(* Logix 5000 AddOnInstructionDefinition export Banner_IOLM_T_v2_2; software revision 32.00 *)

TYPE Banner_IOL_Port_v2 :   // UDT that has all of the data items necessary to communicate with a specific Port on a IO-Link Master
STRUCT
   Port_Controlled : INT;   // Each bit represents a port on an IO-Link Master. Set to 1 to tell AOI to control that port.
   Port_Activate : INT;   // Each bit represents a port on an IO-Link Master. When ON that port will process any commands in queue.
   Port_Read : INT;   // Each bit represents a port on an IO-Link Master. Used to determine when device AOI has requested a Read command.
   Port_Write : INT;   // Each bit represents a port on an IO-Link Master. Used to determine when device AOI has requested a Write command.
   Port_RW_Complete : INT;   // Each bit represents a port on an IO-Link Master. Tells device AOI that Read or Write request has been completed.
   Port_Device_Read : INT;
   Data_Transfer : SINT[70];   // Array to transfer data from IO-Master to device AOIs.
END_STRUCT
END_TYPE

TYPE Banner_IOLM_EL_v2 :   // Error Log for Messages to IOLM.
STRUCT
   RW : SINT;   // 0 = Read, 1 = Write.
   Port : SINT;   // Port number that generated error.
   Index : SINT;   // IO-Link Index for generated error.
END_STRUCT
END_TYPE

TYPE Banner_IOLM_v2 :   // UDT to control IO-Link Masters.
STRUCT
   Message_Source_Data : SINT[70];   // Array used to generate the source data for an Explicit Message
   Message_Destination_Data : SINT[70];   // Array that stores the data from the IO-Link sensor for an Explicit Message.
   Error_Log : Banner_IOLM_EL_v2[10];
   Error_Write_Retry : BOOL;
   Num_Error_MSGS : DINT;
   IO_Link_Master_Busy : BOOL;   // 0 = While waiting for a command, 1 = Processing command
   AOI_Reset : BOOL;
   Port_Data : Banner_IOL_Port_v2;   // All of the necessary data to work with the various ports of the IO-Link Master.
   Halt_Operation : BOOL;   // When parameter is 1 the AOI is halted as next available time frame.
   AOI_Halted : BOOL;   // AOI is in standby mode until Halt Operation tag is set back to 0.
END_STRUCT
END_TYPE

TYPE IOLRequest :
STRUCT
   Enable_Multiple_Nodes : BOOL; {access None}   // Set to 1 to enable multiple nodes
   ApplicationPath : STRING; {access None}   // Set Path for following IOL Instructions
   Read : BOOL; {access None}   // For internal use to integrate IOLRead and IOWrite with IOLService
   Write : BOOL; {access None}   // For internal use to integrate IOLRead and IOWrite with IOLService
   Reset : BOOL; {access None}   // For internal use to integrate IOLRead and IOWrite with IOLService
   Done : BOOL; {access None}   // For internal use to integrate IOLRead and IOWrite with IOLService
   Error : BOOL; {access None}   // For internal use to integrate IOLRead and IOWrite with IOLService
   Slot : INT; {access None}   // For internal use to integrate IOLRead and IOWrite with IOLService
   Port : INT; {access None}   // For internal use to integrate IOLRead and IOWrite with IOLService
   Index : INT; {access None}   // For internal use to integrate IOLRead and IOWrite with IOLService
   SubIndex : INT; {access None}   // For internal use to integrate IOLRead and IOWrite with IOLService
   Length : INT; {access None}   // For internal use to integrate IOLRead and IOWrite with IOLService
   Handle : INT; {access None}   // For internal use to integrate IOLRead and IOWrite with IOLService
   Status : INT; {access None}   // For internal use to integrate IOLRead and IOWrite with IOLService
   NextHandle : INT; {access None}   // For internal use to integrate IOLRead and IOWrite with IOLService
   ReceiveData : SINT[145]; {access None}   // For internal use to integrate IOLRead and IOWrite with IOLService
   SendData : SINT[145]; {access None}   // For internal use to integrate IOLRead and IOWrite with IOLService
   WriteData : DINT; {access None}   // For internal use to integrate IOLRead and IOWrite with IOLService
   ActivePath : STRING; {access None}   // For internal use to integrate IOLRead and IOWrite with IOLService
END_STRUCT
END_TYPE

ADD_ON_INSTRUCTION IOL_ReadData_T   (* revision 1.2, ExecutePrescan, ExecuteEnableInFalse *)
// Revision note:
// V1_0 Initial Release
// V1_1 Automatic data precision detection
// V1_2 Added multiple EIP node support
// Help:
// IOL_ReadData - used with Turck BL20, BL67, BLC and TBEN IOLink masters to read numeric data from IOLink devices.  Use in conjuction with IOLService AOI which processes all IOL read and write requests.
// Status	Description
// 0	Operation completed successfully
// 	Status = 100 - 102, Ethernet IP MSG instruction errors - check communication parameters
// 100	IOL_SendMSG completed with error, check communication parameters
// 101	IOL_RecevieMSG completed with error, check communication parameters
// 110	IOL_Service Retry Limit exceeded
// 111	Slot specified not an IOLink master
// 	Status = 1000 to 1255, no response from device, connection error
// 1016	Device not connected or Port not configured as IOLink port
// 	Status = 2000 to 2255,  device response indicates error
// 2000	Device error, no details
// 2017	Device error, Index not available
// 2018	Device error, Subindex not available
// 2032	Device error, Service temporarily not available
// 2033	Device error, Service temporarily not available - local control
// 2034	Device error, Service temporarily not available - device control
// 2035	Device error, Index not writeable
// 2048	Device error, Parameter value out of range
// 2049	Device error, Parameter value above limit
// 2050	Device error, Parameter value below limit
// 2051	Device error, Parameter value length overrun (check IOLWrite precision/string length)
// 2052	Device error, Parameter value length underrun (check IOLWrite precision/string length)
// 2053	Device error, Function not available
// 2054	Device error, Function temporarily not available
// 2064	Device error, Parameter set invalid
// 2065	Device error, Inconsistent parameter set
// 2130	Device error, Application not ready
// 	Status = 3000 to 3255,   device response indicates vendor specific error
// 3000	Vendor specific error, no details
// 3001	Vendor specific error, vendor specific error number
// 3255	Vendor specific error, vendor specific error number
// 	Status = 7000 to 7255,  IOL-M Error Codes
// 7000	Unexpected write request instead of read request
// 7001	Decode error
// 7002	Port occupied by another task
// 	Status = 8000 to 8255,  IOL-M Error Codes
// 8000	Timeout when IOL-Ds or IOL-M ports are busy
// 8001	IOL Index out of range
// 8002	Port address greater than maximum
// 8003	Port function not supported
VAR_OUTPUT
   Done : BOOL; {access Read Only, visible}   // IOLRead completed successfully
   Error : BOOL; {access Read Only, visible}   // IOLRead completed with error, check status
   Pending : BOOL; {access Read Only, visible}   // IOLRead waiting to be processed
   Active : BOOL; {access Read Only, visible}   // IOLRead in progress
END_VAR
VAR_IN_OUT
   IOLData : IOLRequest; {required}   // Shared IOL Data Area - must be identical on all requests
END_VAR
VAR_OUTPUT
   DoneCount : DINT; {access Read Only, visible}   // Number of operations completed successfully
   ErrorCount : DINT; {access Read Only, visible}   // Number of operations competed with error
   Status : INT; {access Read Only, visible}   // Status of last IOLRead
END_VAR
VAR_INPUT
   Read : BOOL;   // Rising edge triggers IOLink Read
   Read_Continuous : BOOL;   // Set to trigger IOLink Read repeatedly
END_VAR
VAR_OUTPUT
   ReadData : DINT; {access Read Only, required}   // Data returned from IOLink device
END_VAR
VAR_INPUT
   R_8_Bit : BOOL;   // Indicates data received is 8 bit precision
   R_16_Bit : BOOL;   // Indicates data received is 16 bit precision
   R_32_Bit : BOOL;   // Indicates data received is 32 bit precision
   R_Sign_Extend : BOOL;   // Set to extend 8/16 bit precision data sign bit
   R_Swap_16 : BOOL;   // 16-bit AB->BA, 32-bit ABCD->BADC
   R_Swap_32 : BOOL;   // 32-bit ABCD->DCBA
   R_Swap_All : BOOL;   // 32-bit ABCD->CDBA
END_VAR
VAR
   MyHandle : INT;
   StartupDone : BOOL; {access None}
   Pending_or_Active : BOOL; {access None}
   Read_ONS : BOOL; {access None}
   StartupCount : DINT; {access None}
   ReadSignBit : DINT; {access None}
   ReadRequest : BOOL; {access None}
END_VAR

ROUTINE EnableInFalse   (* ladder *)
END_ROUTINE

ROUTINE Logic   (* ladder *)
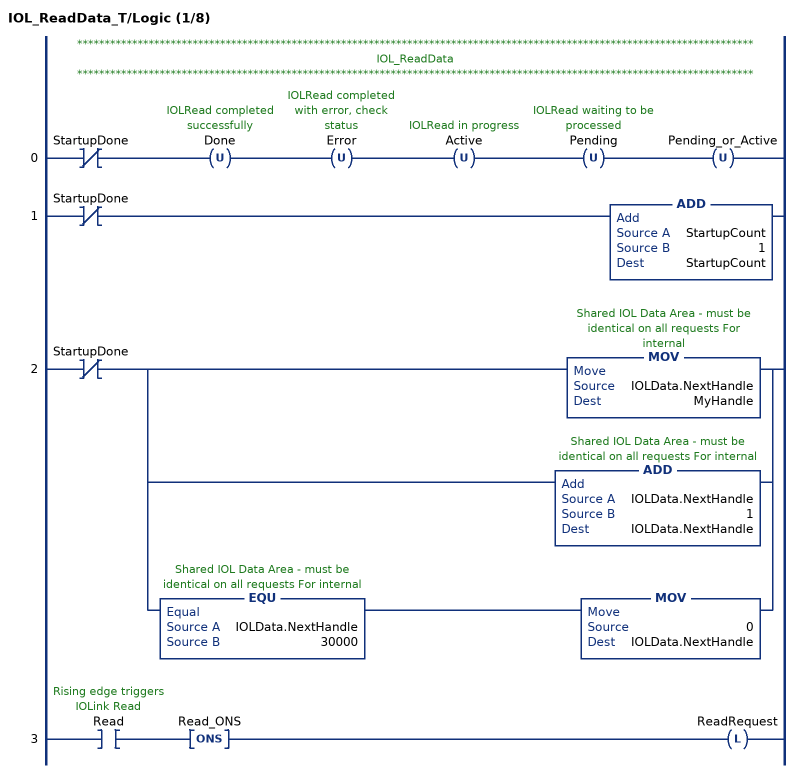
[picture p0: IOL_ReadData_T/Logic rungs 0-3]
   // ***************************************************************************************************************************
   // IOL_ReadData
   // ***************************************************************************************************************************
   0: XIO(StartupDone)OTU(Done)OTU(Error)OTU(Active)OTU(Pending)OTU(Pending_or_Active);
   1: XIO(StartupDone)ADD(StartupCount,1,StartupCount);
   2: XIO(StartupDone)[MOV(IOLData.NextHandle,MyHandle) ,ADD(IOLData.NextHandle,1,IOLData.NextHandle) ,EQU(IOLData.NextHandle,30000) MOV(0,IOLData.NextHandle) ];
   3: XIC(Read)ONS(Read_ONS)OTL(ReadRequest);
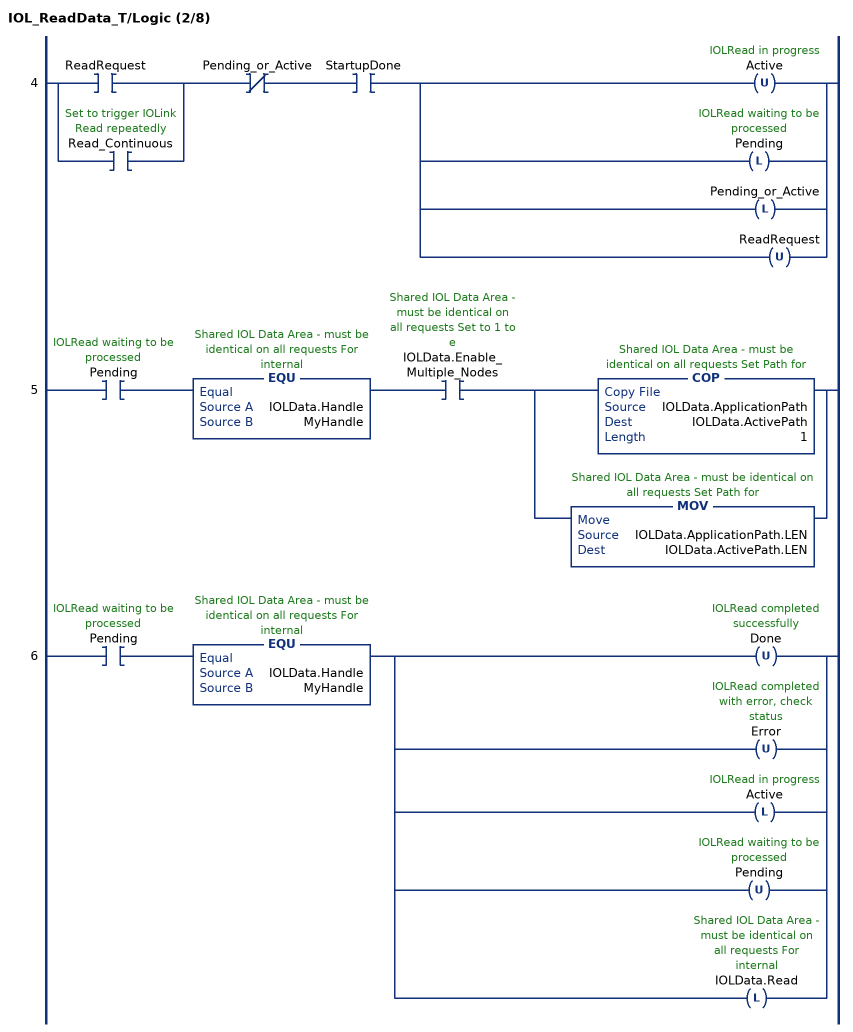
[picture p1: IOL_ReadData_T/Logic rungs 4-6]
   4: [XIC(ReadRequest) ,XIC(Read_Continuous) ]XIO(Pending_or_Active)XIC(StartupDone)[OTU(Active) ,OTL(Pending) ,OTL(Pending_or_Active) ,OTU(ReadRequest) ];
   5: XIC(Pending)EQU(IOLData.Handle,MyHandle)XIC(IOLData.Enable_Multiple_Nodes)[COP(IOLData.ApplicationPath,IOLData.ActivePath,1) ,MOV(IOLData.ApplicationPath.LEN,IOLData.ActivePath.LEN) ];
   6: XIC(Pending)EQU(IOLData.Handle,MyHandle)[OTU(Done) ,OTU(Error) ,OTL(Active) ,OTU(Pending) ,OTL(IOLData.Read) ];
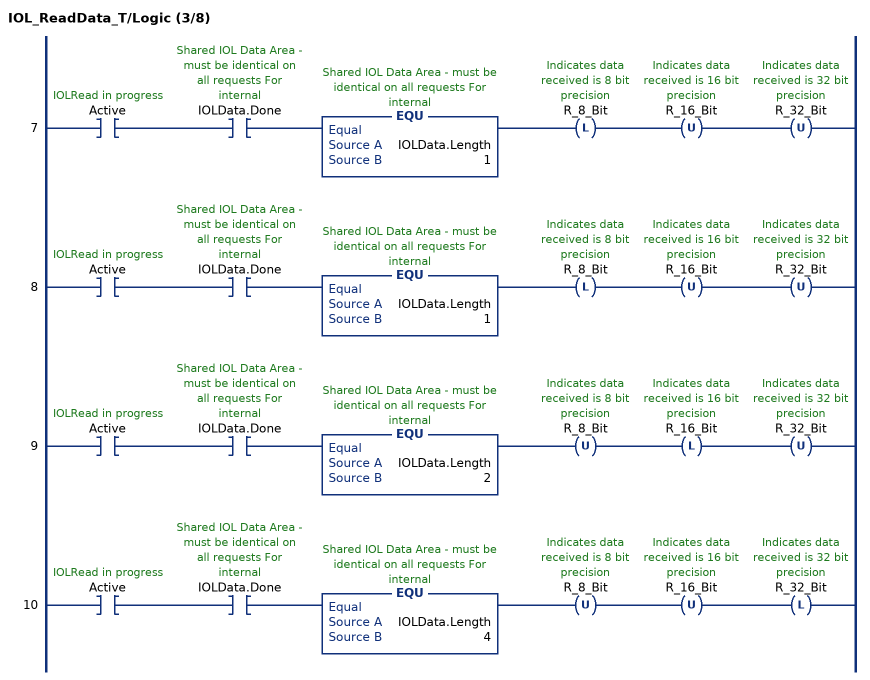
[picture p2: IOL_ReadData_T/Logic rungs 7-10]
   7: XIC(Active)XIC(IOLData.Done)EQU(IOLData.Length,1)OTL(R_8_Bit)OTU(R_16_Bit)OTU(R_32_Bit);
   8: XIC(Active)XIC(IOLData.Done)EQU(IOLData.Length,1)OTL(R_8_Bit)OTU(R_16_Bit)OTU(R_32_Bit);
   9: XIC(Active)XIC(IOLData.Done)EQU(IOLData.Length,2)OTU(R_8_Bit)OTL(R_16_Bit)OTU(R_32_Bit);
   10: XIC(Active)XIC(IOLData.Done)EQU(IOLData.Length,4)OTU(R_8_Bit)OTU(R_16_Bit)OTL(R_32_Bit);
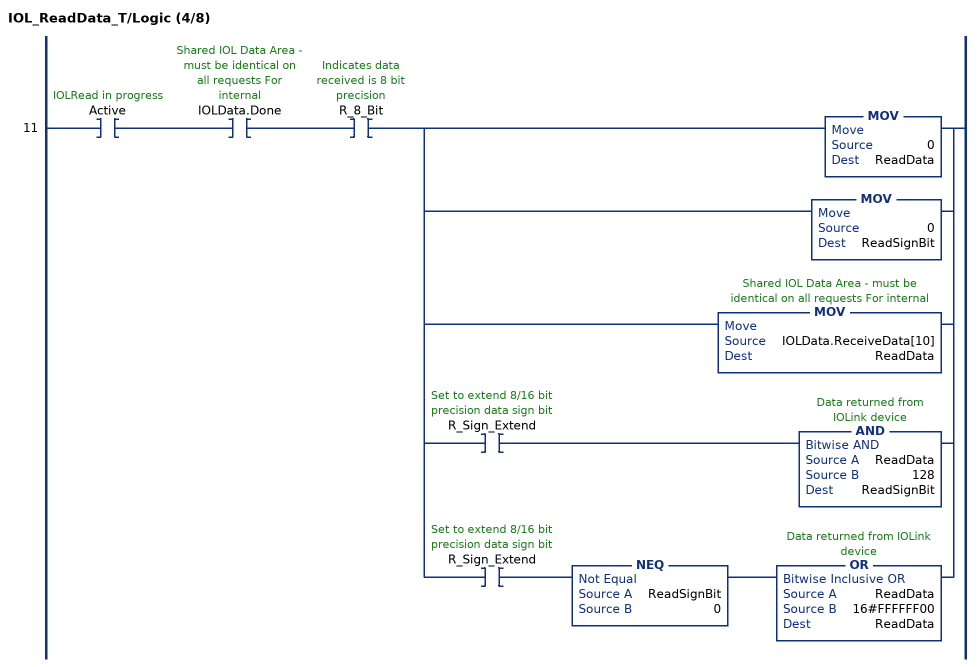
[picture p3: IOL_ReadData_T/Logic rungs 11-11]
   11: XIC(Active)XIC(IOLData.Done)XIC(R_8_Bit)[MOV(0,ReadData) ,MOV(0,ReadSignBit) ,MOV(IOLData.ReceiveData[10],ReadData) ,XIC(R_Sign_Extend) AND(ReadData,128,ReadSignBit) ,XIC(R_Sign_Extend) NEQ(ReadSignBit,0) OR(ReadData,16#FFFFFF00,ReadData) ];
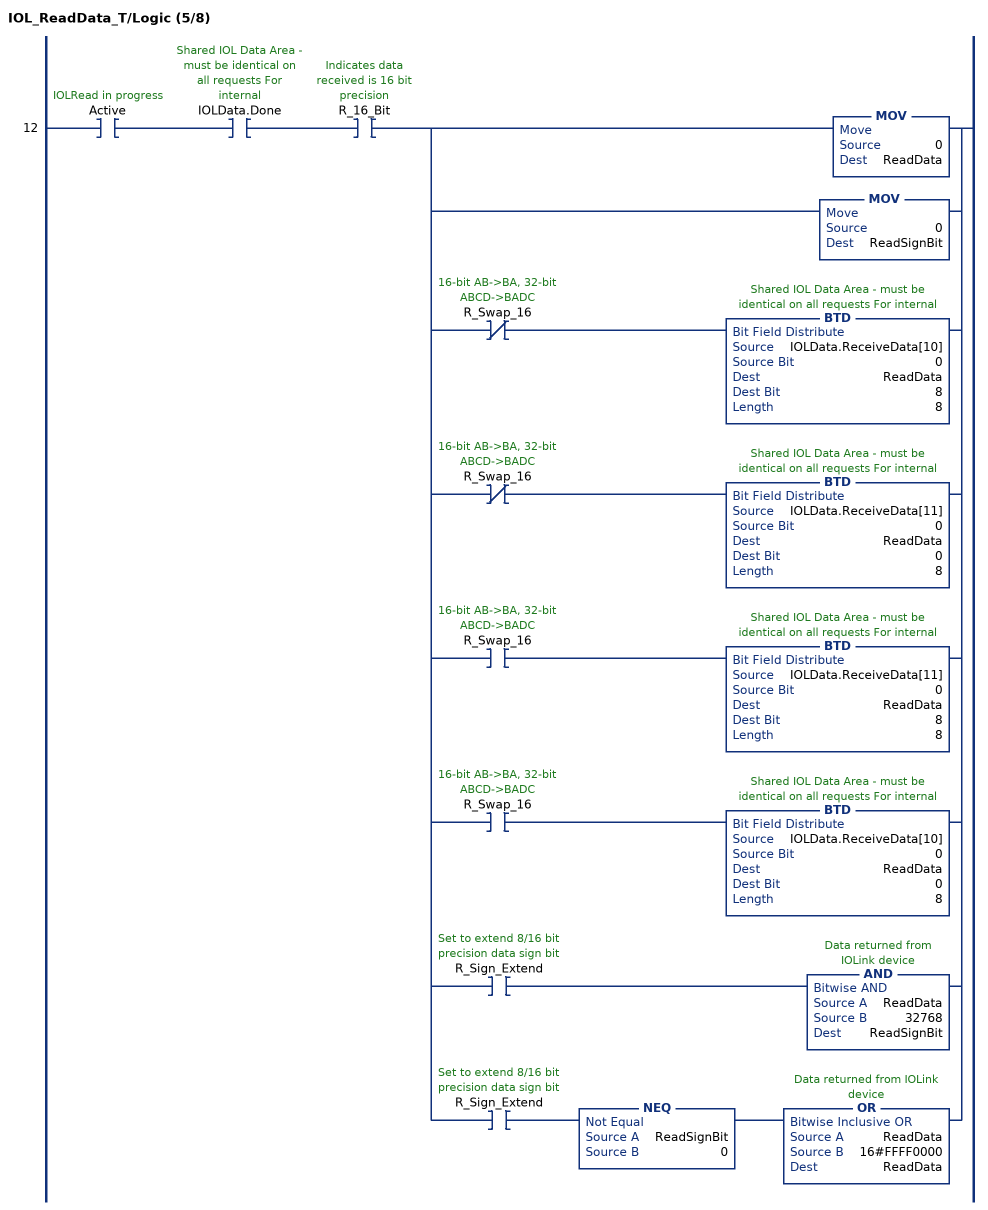
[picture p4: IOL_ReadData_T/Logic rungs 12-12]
   12: XIC(Active)XIC(IOLData.Done)XIC(R_16_Bit)[MOV(0,ReadData) ,MOV(0,ReadSignBit) ,XIO(R_Swap_16) BTD(IOLData.ReceiveData[10],0,ReadData,8,8) ,XIO(R_Swap_16) BTD(IOLData.ReceiveData[11],0,ReadData,0,8) ,XIC(R_Swap_16) BTD(IOLData.ReceiveData[11],0,ReadData,8,8) ,XIC(R_Swap_16) BTD(IOLData.ReceiveData[10],0,ReadData,0,8) ,XIC(R_Sign_Extend) AND(ReadData,32768,ReadSignBit) ,XIC(R_Sign_Extend) NEQ(ReadSignBit,0) OR(ReadData,16#FFFF0000,ReadData) ];
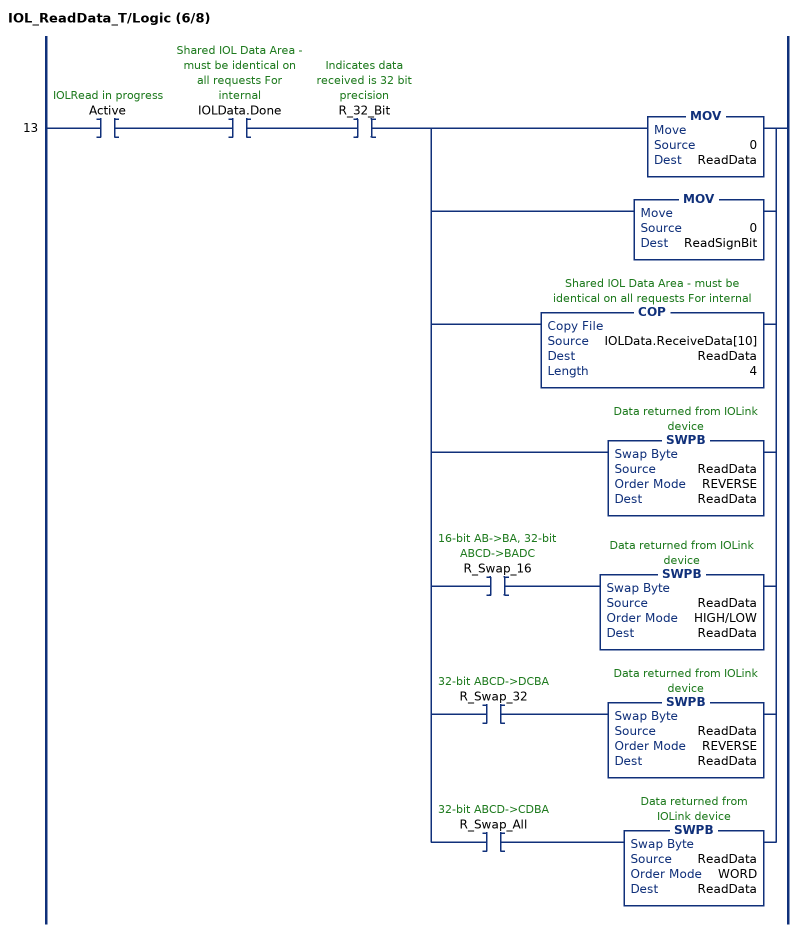
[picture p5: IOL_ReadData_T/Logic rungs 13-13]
   13: XIC(Active)XIC(IOLData.Done)XIC(R_32_Bit)[MOV(0,ReadData) ,MOV(0,ReadSignBit) ,COP(IOLData.ReceiveData[10],ReadData,4) ,SWPB(ReadData,REVERSE,ReadData) ,XIC(R_Swap_16) SWPB(ReadData,HIGH/LOW,ReadData) ,XIC(R_Swap_32) SWPB(ReadData,REVERSE,ReadData) ,XIC(R_Swap_All) SWPB(ReadData,WORD,ReadData) ];
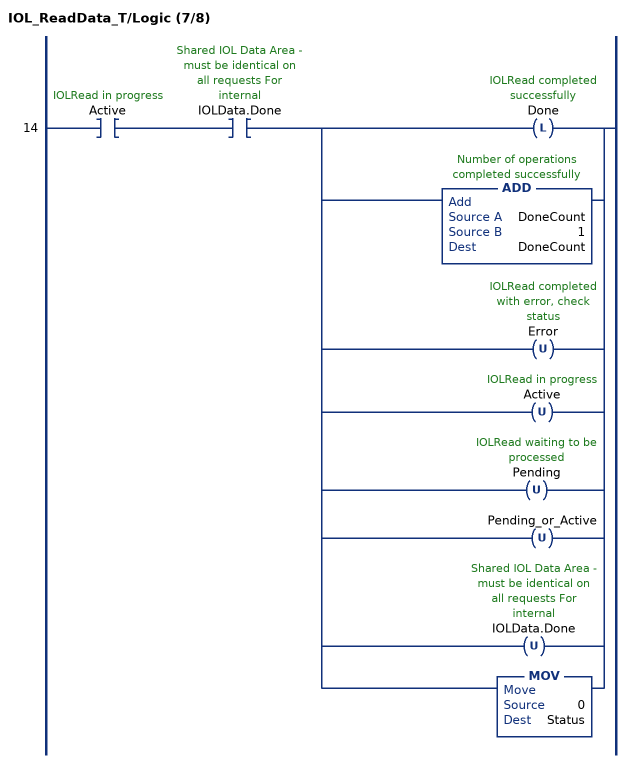
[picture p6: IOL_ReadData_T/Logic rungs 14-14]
   14: XIC(Active)XIC(IOLData.Done)[OTL(Done) ,ADD(DoneCount,1,DoneCount) ,OTU(Error) ,OTU(Active) ,OTU(Pending) ,OTU(Pending_or_Active) ,OTU(IOLData.Done) ,MOV(0,Status) ];
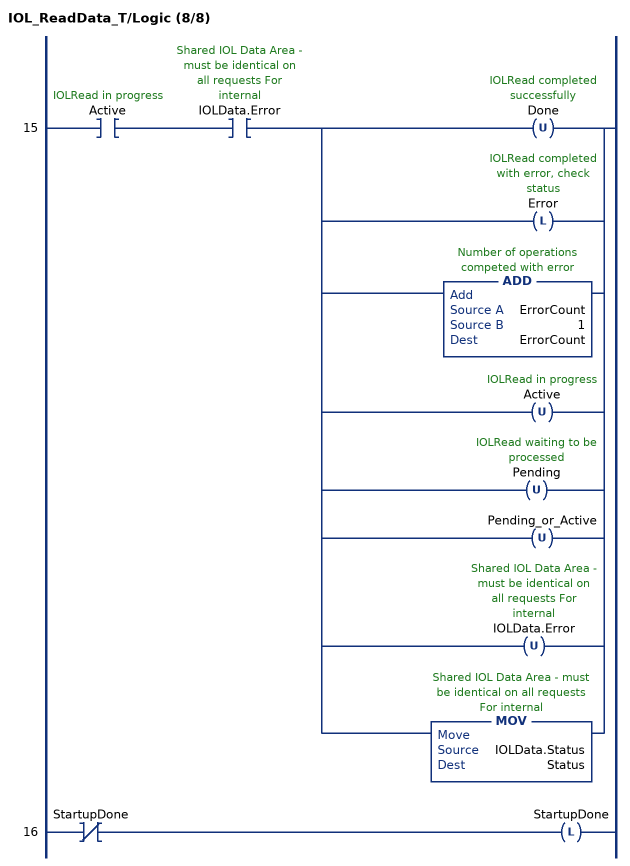
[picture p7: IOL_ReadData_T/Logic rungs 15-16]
   15: XIC(Active)XIC(IOLData.Error)[OTU(Done) ,OTL(Error) ,ADD(ErrorCount,1,ErrorCount) ,OTU(Active) ,OTU(Pending) ,OTU(Pending_or_Active) ,OTU(IOLData.Error) ,MOV(IOLData.Status,Status) ];
   16: XIO(StartupDone)OTL(StartupDone);
END_ROUTINE

ROUTINE Prescan   (* ladder *)
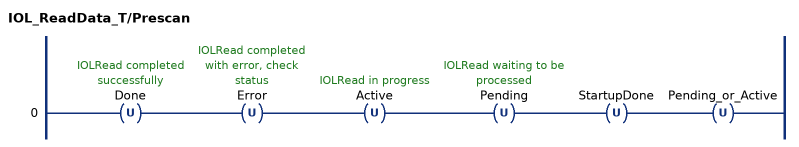
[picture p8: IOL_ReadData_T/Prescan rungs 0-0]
   0: OTU(Done)OTU(Error)OTU(Active)OTU(Pending)OTU(StartupDone)OTU(Pending_or_Active);
END_ROUTINE
END_ADD_ON_INSTRUCTION

ADD_ON_INSTRUCTION Banner_IOLM_T_v2_2   (* revision 2.2, vendor Banner Engineering *)
// AOI that controls a Turck IO-Link Master with Banner devices.
// Revision note:
// Added error handling for read commands.
VAR_IN_OUT
   Message : MESSAGE; {required}   // Message used to gather data from a device plugged into an Allen Bradley IO-Link Master.
   IOLM : Banner_IOLM_v2; {required}
   IOLData : IOLRequest; {required}   // Structure that interfaces with Turck AOI.
   IOL_ReadData : IOL_ReadData_T; {required}   // Structure that interfaces with Turck AOI.
END_VAR
VAR_INPUT
   Slot : INT; {required}
END_VAR
VAR
   Lock : DINT; {access None}
   Disable_Timer : BOOL; {access None}
   Byte_Length : SINT; {access None}
   Current_Port : INT; {access None}   // Current port to communicate with via the IO-Link Master.
   Array_Index : DINT; {access None}
   Data_Index : DINT; {access None}
   ReadData : DINT; {access None}
   Message_Timer : TIMER := (PRE := 1000); {access None}
   TEMP : DINT[10]; {access None}
   Error_Index : DINT; {access None}
   Message_Timer2 : TIMER := (PRE := 5000); {access None}
   Temp_Index : INT; {access None}
END_VAR

ROUTINE Logic   (* ladder *)
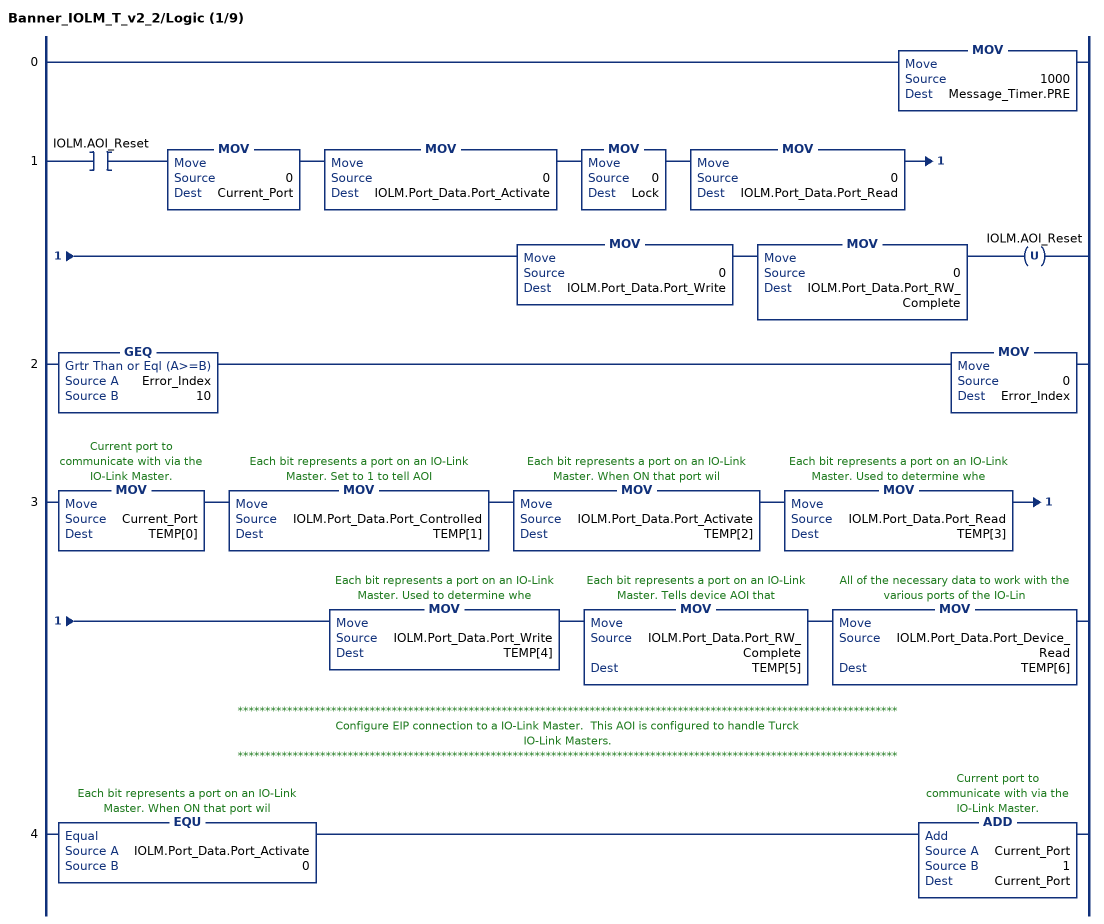
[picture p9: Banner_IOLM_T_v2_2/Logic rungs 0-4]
   0: MOV(1000,Message_Timer.PRE);
   1: XIC(IOLM.AOI_Reset)MOV(0,Current_Port)MOV(0,IOLM.Port_Data.Port_Activate)MOV(0,Lock)MOV(0,IOLM.Port_Data.Port_Read)MOV(0,IOLM.Port_Data.Port_Write)MOV(0,IOLM.Port_Data.Port_RW_Complete)OTU(IOLM.AOI_Reset);
   2: GEQ(Error_Index,10)MOV(0,Error_Index);
   3: MOV(Current_Port,TEMP[0])MOV(IOLM.Port_Data.Port_Controlled,TEMP[1])MOV(IOLM.Port_Data.Port_Activate,TEMP[2])MOV(IOLM.Port_Data.Port_Read,TEMP[3])MOV(IOLM.Port_Data.Port_Write,TEMP[4])MOV(IOLM.Port_Data.Port_RW_Complete,TEMP[5])MOV(IOLM.Port_Data.Port_Device_Read,TEMP[6]);
   // ************************************************************************************************************************
   // Configure EIP connection to a IO-Link Master.  This AOI is configured to handle Turck
   // IO-Link Masters.
   // ************************************************************************************************************************
   4: EQU(IOLM.Port_Data.Port_Activate,0)ADD(Current_Port,1,Current_Port);
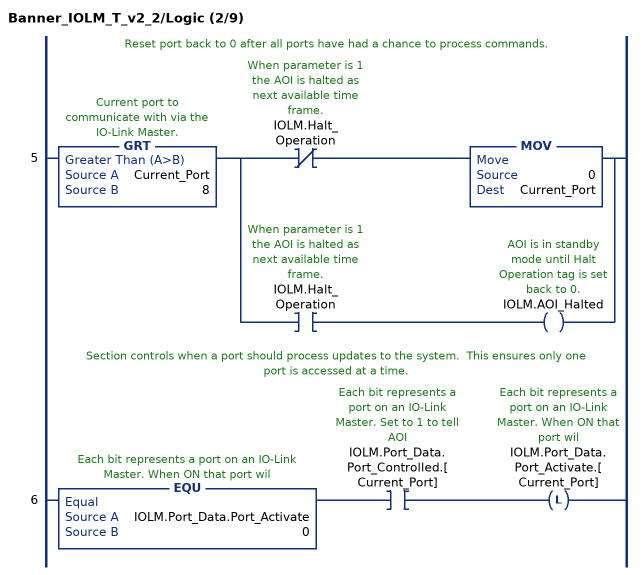
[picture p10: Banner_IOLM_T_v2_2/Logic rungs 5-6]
   // Reset port back to 0 after all ports have had a chance to process commands.
   5: GRT(Current_Port,8)[XIO(IOLM.Halt_Operation) MOV(0,Current_Port) ,XIC(IOLM.Halt_Operation) OTE(IOLM.AOI_Halted) ];
   // Section controls when a port should process updates to the system.  This ensures only one port is accessed at a time.
   6: EQU(IOLM.Port_Data.Port_Activate,0)XIC(IOLM.Port_Data.Port_Controlled.[Current_Port])OTL(IOLM.Port_Data.Port_Activate.[Current_Port]);
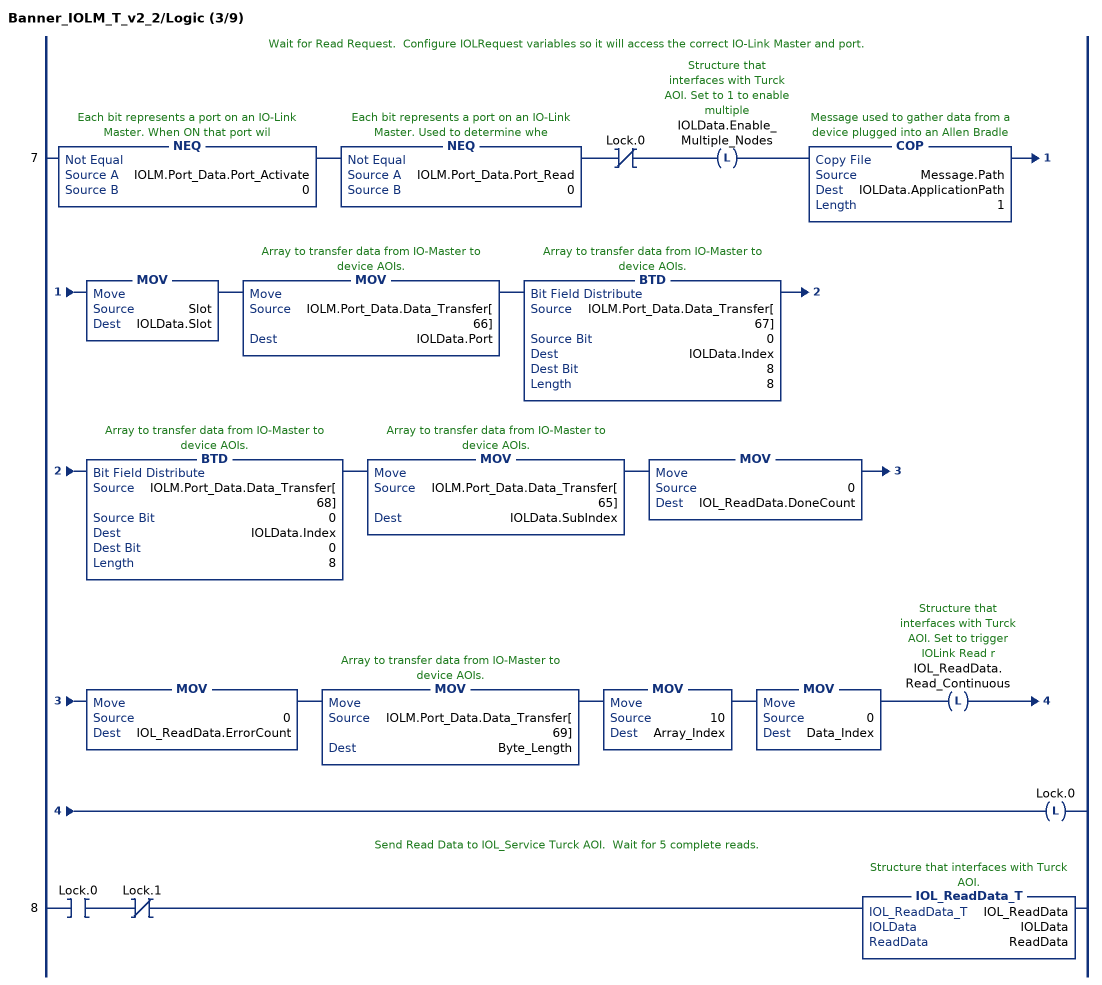
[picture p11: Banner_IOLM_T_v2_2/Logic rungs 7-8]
   // Wait for Read Request.  Configure IOLRequest variables so it will access the correct IO-Link Master and port.
   7: NEQ(IOLM.Port_Data.Port_Activate,0)NEQ(IOLM.Port_Data.Port_Read,0)XIO(Lock.0)OTL(IOLData.Enable_Multiple_Nodes)COP(Message.Path,IOLData.ApplicationPath,1)MOV(Slot,IOLData.Slot)MOV(IOLM.Port_Data.Data_Transfer[66],IOLData.Port)BTD(IOLM.Port_Data.Data_Transfer[67],0,IOLData.Index,8,8)BTD(IOLM.Port_Data.Data_Transfer[68],0,IOLData.Index,0,8)MOV(IOLM.Port_Data.Data_Transfer[65],IOLData.SubIndex)MOV(0,IOL_ReadData.DoneCount)MOV(0,IOL_ReadData.ErrorCount)MOV(IOLM.Port_Data.Data_Transfer[69],Byte_Length)MOV(10,Array_Index)MOV(0,Data_Index)OTL(IOL_ReadData.Read_Continuous)OTL(Lock.0);
   // Send Read Data to IOL_Service Turck AOI.  Wait for 5 complete reads.
   8: XIC(Lock.0)XIO(Lock.1)IOL_ReadData_T(IOL_ReadData,IOLData,ReadData);
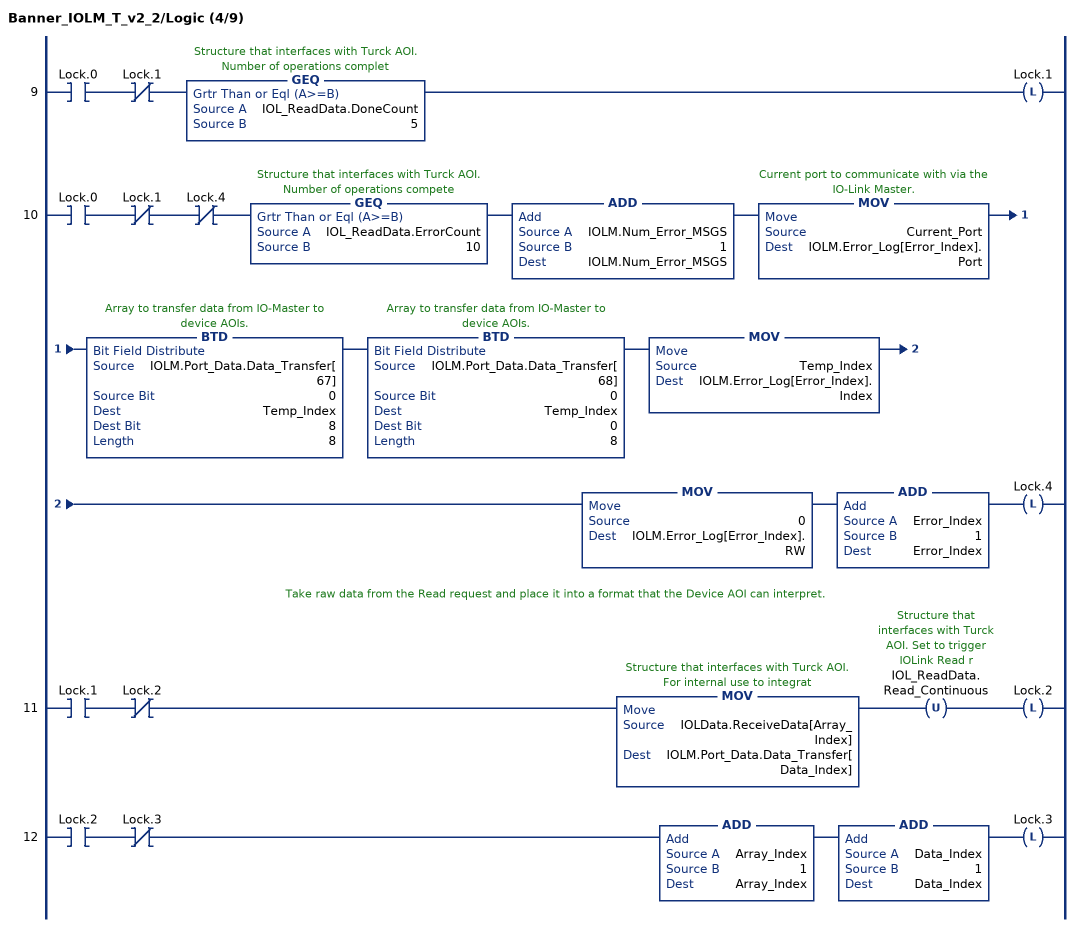
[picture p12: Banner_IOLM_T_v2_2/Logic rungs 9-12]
   9: XIC(Lock.0)XIO(Lock.1)GEQ(IOL_ReadData.DoneCount,5)OTL(Lock.1);
   10: XIC(Lock.0)XIO(Lock.1)XIO(Lock.4)GEQ(IOL_ReadData.ErrorCount,10)ADD(IOLM.Num_Error_MSGS,1,IOLM.Num_Error_MSGS)MOV(Current_Port,IOLM.Error_Log[Error_Index].Port)BTD(IOLM.Port_Data.Data_Transfer[67],0,Temp_Index,8,8)BTD(IOLM.Port_Data.Data_Transfer[68],0,Temp_Index,0,8)MOV(Temp_Index,IOLM.Error_Log[Error_Index].Index)MOV(0,IOLM.Error_Log[Error_Index].RW)ADD(Error_Index,1,Error_Index)OTL(Lock.4);
   // Take raw data from the Read request and place it into a format that the Device AOI can interpret.
   11: XIC(Lock.1)XIO(Lock.2)MOV(IOLData.ReceiveData[Array_Index],IOLM.Port_Data.Data_Transfer[Data_Index])OTU(IOL_ReadData.Read_Continuous)OTL(Lock.2);
   12: XIC(Lock.2)XIO(Lock.3)ADD(Array_Index,1,Array_Index)ADD(Data_Index,1,Data_Index)OTL(Lock.3);
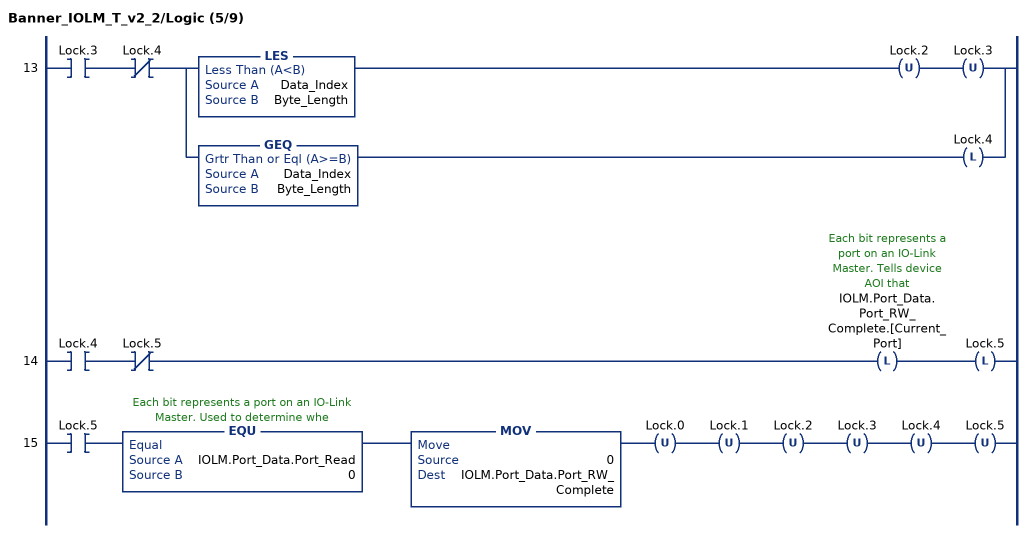
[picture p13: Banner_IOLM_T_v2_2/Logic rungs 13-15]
   13: XIC(Lock.3)XIO(Lock.4)[LES(Data_Index,Byte_Length) OTU(Lock.2) OTU(Lock.3) ,GEQ(Data_Index,Byte_Length) OTL(Lock.4) ];
   14: XIC(Lock.4)XIO(Lock.5)OTL(IOLM.Port_Data.Port_RW_Complete.[Current_Port])OTL(Lock.5);
   15: XIC(Lock.5)EQU(IOLM.Port_Data.Port_Read,0)MOV(0,IOLM.Port_Data.Port_RW_Complete)OTU(Lock.0)OTU(Lock.1)OTU(Lock.2)OTU(Lock.3)OTU(Lock.4)OTU(Lock.5);
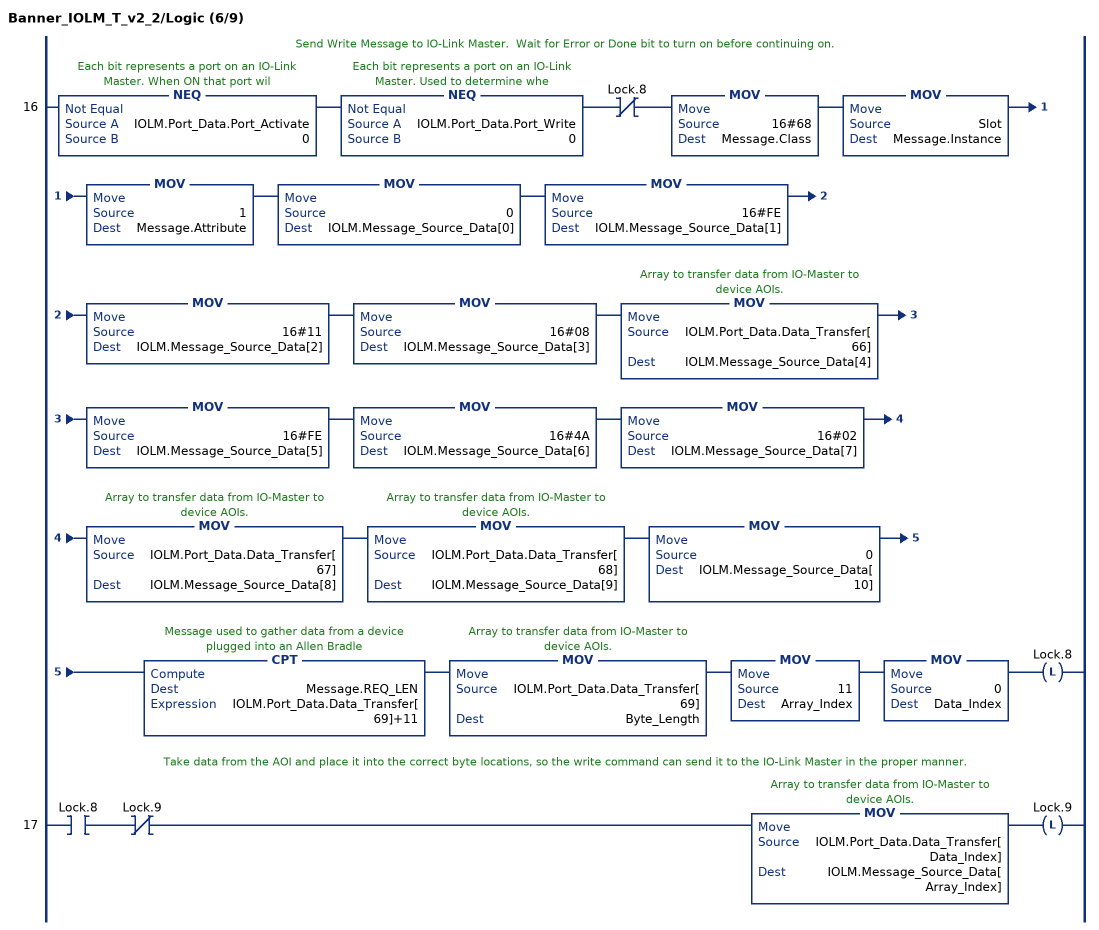
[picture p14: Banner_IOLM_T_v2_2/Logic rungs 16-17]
   // Send Write Message to IO-Link Master.  Wait for Error or Done bit to turn on before continuing on.
   16: NEQ(IOLM.Port_Data.Port_Activate,0)NEQ(IOLM.Port_Data.Port_Write,0)XIO(Lock.8)MOV(16#68,Message.Class)MOV(Slot,Message.Instance)MOV(1,Message.Attribute)MOV(0,IOLM.Message_Source_Data[0])MOV(16#FE,IOLM.Message_Source_Data[1])MOV(16#11,IOLM.Message_Source_Data[2])MOV(16#08,IOLM.Message_Source_Data[3])MOV(IOLM.Port_Data.Data_Transfer[66],IOLM.Message_Source_Data[4])MOV(16#FE,IOLM.Message_Source_Data[5])MOV(16#4A,IOLM.Message_Source_Data[6])MOV(16#02,IOLM.Message_Source_Data[7])MOV(IOLM.Port_Data.Data_Transfer[67],IOLM.Message_Source_Data[8])MOV(IOLM.Port_Data.Data_Transfer[68],IOLM.Message_Source_Data[9])MOV(0,IOLM.Message_Source_Data[10])CPT(Message.REQ_LEN,IOLM.Port_Data.Data_Transfer[69]+11)MOV(IOLM.Port_Data.Data_Transfer[69],Byte_Length)MOV(11,Array_Index)MOV(0,Data_Index)OTL(Lock.8);
   // Take data from the AOI and place it into the correct byte locations, so the write command can send it to the IO-Link Master in the proper manner.
   17: XIC(Lock.8)XIO(Lock.9)MOV(IOLM.Port_Data.Data_Transfer[Data_Index],IOLM.Message_Source_Data[Array_Index])OTL(Lock.9);
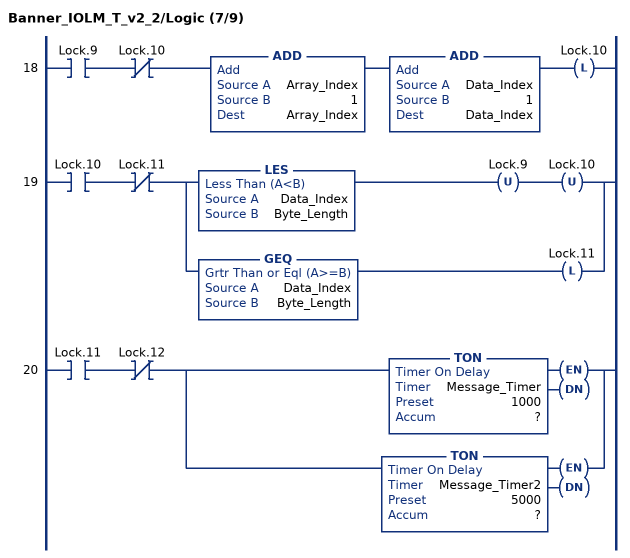
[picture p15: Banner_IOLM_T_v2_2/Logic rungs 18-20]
   18: XIC(Lock.9)XIO(Lock.10)ADD(Array_Index,1,Array_Index)ADD(Data_Index,1,Data_Index)OTL(Lock.10);
   19: XIC(Lock.10)XIO(Lock.11)[LES(Data_Index,Byte_Length) OTU(Lock.9) OTU(Lock.10) ,GEQ(Data_Index,Byte_Length) OTL(Lock.11) ];
   20: XIC(Lock.11)XIO(Lock.12)[TON(Message_Timer,?,?) ,TON(Message_Timer2,?,?) ];
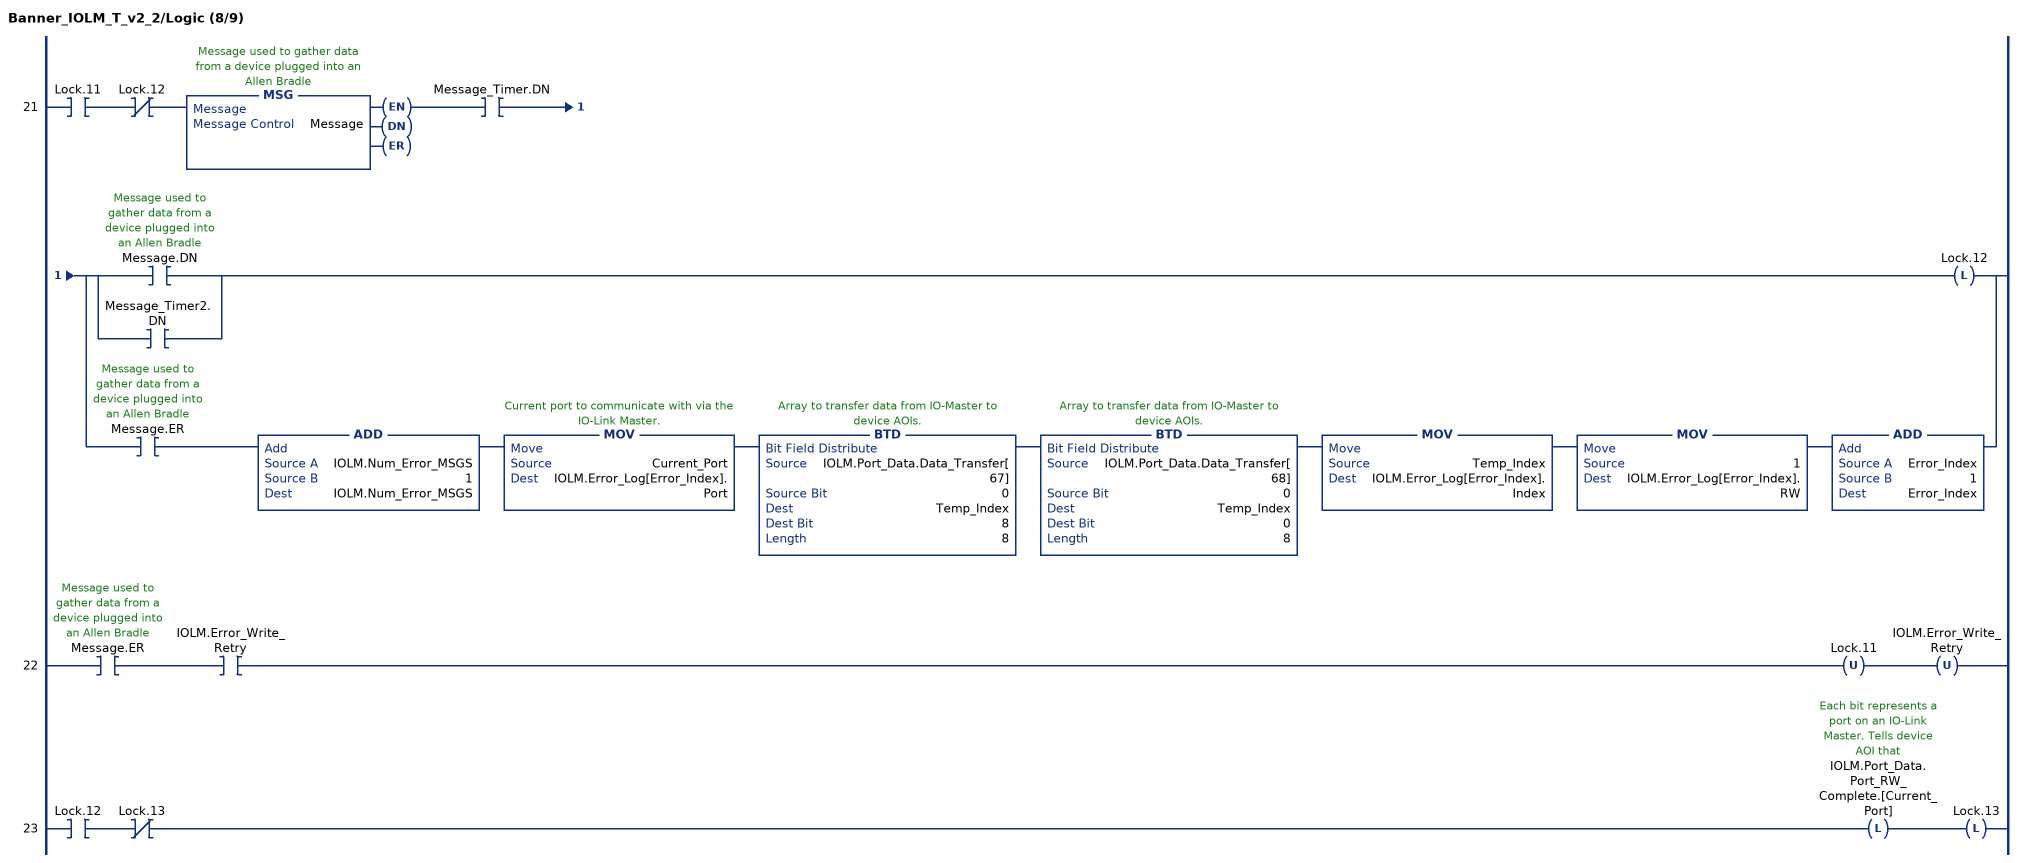
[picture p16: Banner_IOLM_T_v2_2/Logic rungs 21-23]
   21: XIC(Lock.11)XIO(Lock.12)MSG(Message)XIC(Message_Timer.DN)[[XIC(Message.DN) ,XIC(Message_Timer2.DN) ] OTL(Lock.12) ,XIC(Message.ER) ADD(IOLM.Num_Error_MSGS,1,IOLM.Num_Error_MSGS) MOV(Current_Port,IOLM.Error_Log[Error_Index].Port) BTD(IOLM.Port_Data.Data_Transfer[67],0,Temp_Index,8,8) BTD(IOLM.Port_Data.Data_Transfer[68],0,Temp_Index,0,8) MOV(Temp_Index,IOLM.Error_Log[Error_Index].Index) MOV(1,IOLM.Error_Log[Error_Index].RW) ADD(Error_Index,1,Error_Index) ];
   22: XIC(Message.ER)XIC(IOLM.Error_Write_Retry)OTU(Lock.11)OTU(IOLM.Error_Write_Retry);
   23: XIC(Lock.12)XIO(Lock.13)OTL(IOLM.Port_Data.Port_RW_Complete.[Current_Port])OTL(Lock.13);
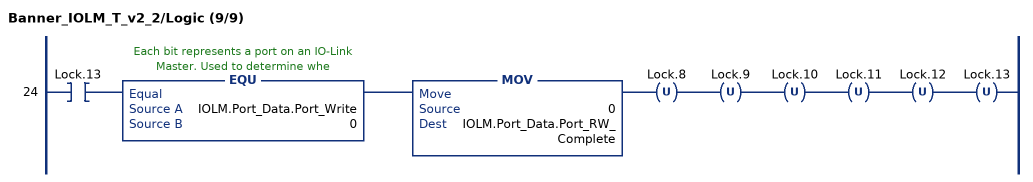
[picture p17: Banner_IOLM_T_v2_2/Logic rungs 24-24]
   24: XIC(Lock.13)EQU(IOLM.Port_Data.Port_Write,0)MOV(0,IOLM.Port_Data.Port_RW_Complete)OTU(Lock.8)OTU(Lock.9)OTU(Lock.10)OTU(Lock.11)OTU(Lock.12)OTU(Lock.13);
END_ROUTINE
END_ADD_ON_INSTRUCTION
